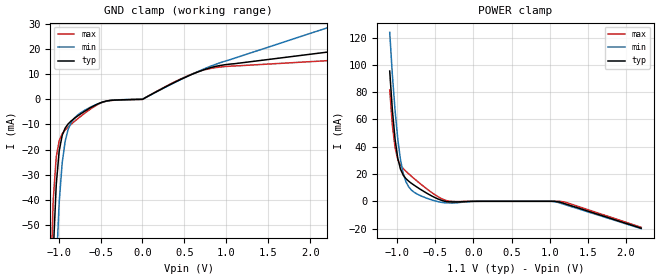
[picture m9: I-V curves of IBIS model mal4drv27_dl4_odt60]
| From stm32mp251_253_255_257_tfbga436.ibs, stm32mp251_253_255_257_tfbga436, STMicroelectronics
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[Model] mal4drv27_dl4_odt60
Model_type   Input
Polarity   Non-Inverting
Enable   Active-High
C_comp   1.569pF   1.545pF   1.591pF
C_comp_power_clamp   881.669fF   863.537fF   898.523fF
C_comp_gnd_clamp 584.387fF   579.583fF   604.741fF
Vinh = 435.000mV
Vinl = 315.000mV
[Model Spec]
D_overshoot_ampl_h 0.3 NA   NA
D_overshoot_ampl_l 0.3 NA   NA
D_overshoot_area_l 100.000m NA   NA
D_overshoot_area_h 100.000m NA   NA
[Receiver Thresholds]
Vth = 375.000mV
Vth_min = 361.000mV
Vth_max = 399.000mV
Vinh_ac = 600.000mV
Vinh_dc = 600.000mV
Vinl_ac = -600.000mV
Vinl_dc = -600.000mV
Tslew_ac = 5.000ns
Threshold_sensitivity = 0.5
Reference_supply Power_clamp_ref
[Temperature Range]   25.000   125.000   -40.000
[Voltage Range]   1.100V   1.060V   1.170V
[GND Clamp Reference]   0.00V   0.00V   0.00V
[C Comp Corner]
| variable   typ   min   max
C_comp 1.569pF   1.545pF   1.591pF
C_comp_pullup 881.669fF   863.537fF   898.523fF
C_comp_pulldown 584.387fF   604.741fF   579.583fF
[POWER Clamp Reference]   1.100V   1.060V   1.170V
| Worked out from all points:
|   GND clamp passes 1 mA (typ) near -0.47 V on its own axis
|   POWER clamp passes 1 mA (typ) near -0.43 V on its own axis
[GND Clamp]
-1.099V   -108.8mA   -166.3mA   -78.76mA
-1.064V   -61.35mA   -108.8mA   -40.13mA
-1.028V   -33.98mA   -67.54mA   -22.97mA
-992.7mV  -20.54mA   -40.97mA   -16.46mA
-957.3mV  -14.41mA   -25.37mA   -13.74mA
-921.8mV  -11.46mA   -16.72mA   -12.2mA
-886.4mV  -9.812mA   -11.99mA   -11.02mA
-709.1mV  -5.201mA   -4.779mA   -6.073mA
-425.5mV  -653.2uA   -711.4uA   -699.1uA
-1.5uV    -14.73uA   -9.993uA   -18.37uA
780mV     12.28mA    12.74mA    12.06mA
2.198V    18.76mA    28.4mA     15.36mA
[Power Clamp]
-1.098V   95.44mA    123.8mA    81.64mA
-1.063V   66.55mA    92.39mA    55.46mA
-1.027V   45.1mA     65.96mA    39.06mA
-991.8mV  31.29mA    45.25mA    30.67mA
-956.4mV  23.46mA    30.33mA    26.52mA
-885.5mV  16.61mA    14.34mA    21.98mA
-779.1mV  11.83mA    6.677mA    16.7mA
-495.5mV  2.468mA    165.5uA    4.447mA
-318.2mV  -379.8uA   -1.218mA   45.31uA
1.029V    -5.783nA   -39.57uA   -731.1pA
1.206V    -1.898mA   -2.568mA   -657.2uA
2.199V    -19.75mA   -20.05mA   -19.1mA
